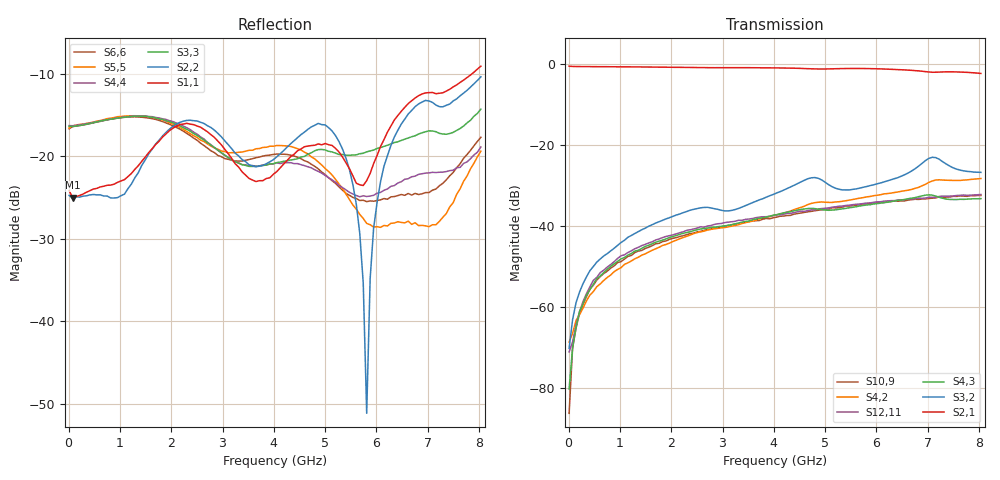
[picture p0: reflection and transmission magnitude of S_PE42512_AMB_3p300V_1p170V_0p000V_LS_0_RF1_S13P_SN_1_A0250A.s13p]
! Device ID: PE42512
! File Path: z:\PE42512\TE_GND_Post_Char_S-Param\All Parts\AMB\3p300\LS_0_RF1\PE42512_AMB_3p300V_1p170V_0p000V_LS_0_RF1_S13P_SN_1_A0250A.s13p
! Serial: 1
! Lot: A0250A
! Temp: AMB
! VDD: 3.300
! VSS: 0.000
! Control_Hi: 1.170
! Control_Lo: 0.000
! Logic State: LS_0_RF1
! Port 1:
! Port 2:
! Port 3:
! Port 4:
! Port 5:
! Port 6:
! Port 7:
! Port 8:
! Port 9:
! Port 10:
! Port 11:
! Port 12:
! Port 13:
! ThroughPath:1-2
! IDD: 0.0001060619
! ISS/IDD2: 1.334e-007
! IDMM3/IDD3: -2.231e-007
! Comment:
#  Hz  S  RI  R  50
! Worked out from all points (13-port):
!   120 points, 10 MHz to 8.037 GHz, reference 50 ohm
!   strongest paths, dB at 10 MHz, 2.034 GHz, 4.057 GHz, 6.08 GHz, 8.037 GHz:
!     S2,1: -0.6, -0.9, -1.1, -1.3, -2.4
!     S3,2: -70.3, -37.7, -31.9, -29.4, -26.8
!     S4,3: -80.3, -42.6, -37.3, -34.4, -33.3
!     S12,11: -71.1, -42.2, -37.3, -34.1, -32.3
!     S4,2: -68.7, -43.9, -37.3, -32.3, -28.3
!     S10,9: -86.3, -43.1, -37.9, -34.2, -32.5
!   lowest |S11| = -25.0 dB at 77.45 MHz (marker M1), VSWR 1.12, Z = 55.9 - j0.421 ohm
!   |S11| at or under -10 dB: start of sweep to 7.861 GHz
